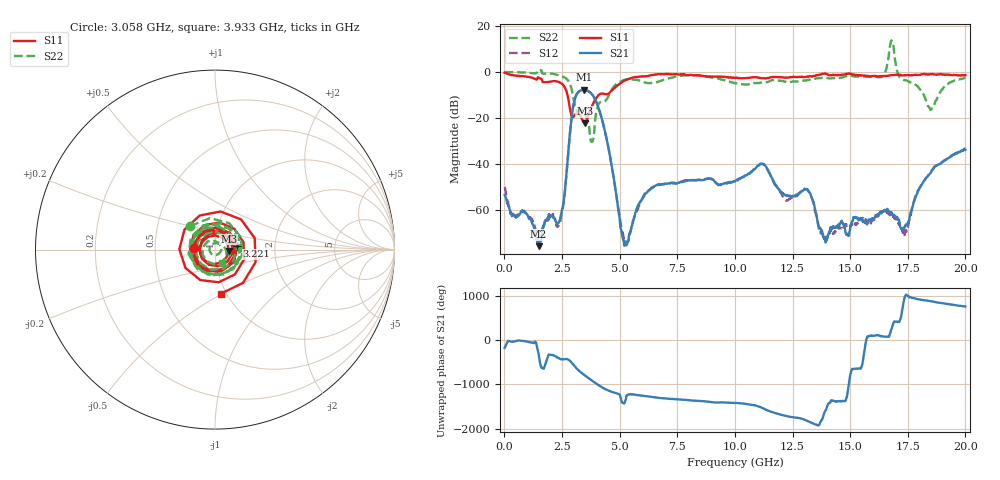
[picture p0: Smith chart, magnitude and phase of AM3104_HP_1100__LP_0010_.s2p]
!Created with skrf (http://scikit-rf.org).
# Hz S RI R 50.0
!freq ReS11 ImS11 ReS21 ImS21 ReS12 ImS12 ReS22 ImS22
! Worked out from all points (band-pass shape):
!   1601 points, 10 MHz to 20 GHz, reference 50 ohm
!   highest |S21| = -7.74 dB at 3.446 GHz (marker M1); lowest = -75.5 dB at 1.484 GHz (marker M2)
!   |S21| within 3 dB of the highest: 3.09 GHz to 3.874 GHz (783.9 MHz wide, 22.5 % of centre)
!   lowest |S11| = -22.3 dB at 3.483 GHz (marker M3), VSWR 1.17, Z = 58.2 - j0.832 ohm
!   |S11| at or under -10 dB: 2.737 GHz to 4.087 GHz (1.35 GHz wide, 39.6 % of centre)
!   |S22| runs from -30.3 to 13.6 dB; largest |S21 - S12| = 0.013
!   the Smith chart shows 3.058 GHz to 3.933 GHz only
!   S11 on the Smith chart (normalised r, x): 3.058 GHz: 0.79, +0.02; 3.221 GHz: 1.27, +0.05; 3.933 GHz: 0.94, -0.49
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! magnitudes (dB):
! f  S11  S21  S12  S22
! 10 MHz  -0.4  -53.3  -49.8  -0.1
! 1.484 GHz  -2.5  -75.5  -73.4  0.8
! 2.434 GHz  -4.8  -62.9  -65.0  -1.7
! 3.058 GHz  -18.5  -11.7  -11.7  -14.4
! 3.221 GHz  -18.2  -8.6  -8.7  -17.0
! 3.346 GHz  -20.0  -7.9  -8.0  -16.5
! 3.446 GHz  -22.0  -7.7  -7.8  -17.9
! 3.483 GHz  -22.3  -7.8  -7.8  -18.4
! 3.796 GHz  -14.7  -9.6  -9.7  -30.3
! 3.933 GHz  -12.1  -11.8  -11.9  -21.5
! 5.22 GHz  -3.7  -74.6  -74.5  -3.4
! 6.682 GHz  -1.0  -48.7  -49.1  -4.2
! 10.01 GHz  -2.6  -47.4  -47.5  -4.9
! 11.18 GHz  -2.8  -39.7  -39.9  -4.6
! 12.19 GHz  -2.5  -53.5  -55.5  -4.3
! 13.34 GHz  -2.0  -54.6  -54.6  -3.2
! 13.92 GHz  -0.6  -73.2  -71.5  -2.4
! 16.35 GHz  -1.8  -60.5  -61.2  -2.3
! 16.68 GHz  -1.5  -60.4  -61.7  7.1
! 17.39 GHz  -1.4  -66.5  -69.2  -3.6
! 18.48 GHz  -0.9  -43.9  -43.8  -16.3
! 20 GHz  -1.4  -33.7  -33.1  -2.7
